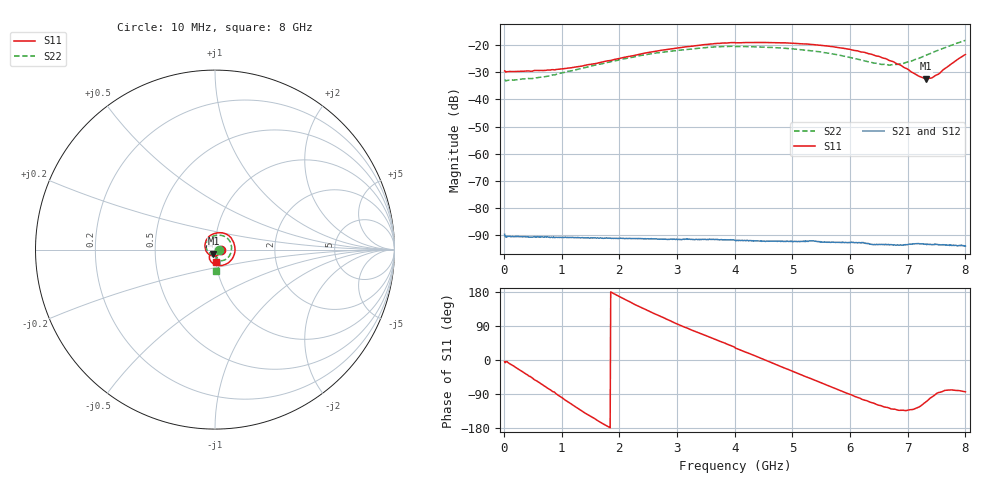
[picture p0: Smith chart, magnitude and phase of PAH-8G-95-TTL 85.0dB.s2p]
! MTS Systemtechnik GmbH
! S-Parameters
! Model: PAH-8G/95-TTL
! Attenuation Step: 85.0dB
! Rohde & Schwarz ZVB8 2Ports - Version 4.11 - 1145.1010k08 SN: 100119
! S2P File Measurements:
! S11 S21 S12 S22
# HZ  S  DB  R  50.00
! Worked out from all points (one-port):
!   800 points, 10 MHz to 8 GHz, reference 50 ohm
!   lowest |S11| = -32.3 dB at 7.32 GHz (marker M1), VSWR 1.05, Z = 49.1 - j2.23 ohm
!   |S11| at or under -10 dB: start of sweep to end of sweep
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1e7  -29.49 -3.7  -89.57 -1.8  -89.72 0.8  -32.75 -5.0
2e8  -29.70 -19.4  -90.45 -28.3  -90.44 -28.0  -32.80 -23.8
6.8e8  -29.35 -66.5  -90.59 -94.7  -90.57 -94.8  -31.70 -79.9
1.02e9  -28.76 -101.1  -90.67 -141.3  -90.71 -141.3  -30.18 -117.2
1.35e9  -27.72 -134.8  -90.86 173.2  -90.80 173.1  -28.55 -149.8
2.05e9  -24.64 163.6  -91.12 76.8  -91.16 76.9  -25.16 151.5
2.68e9  -22.09 117.0  -91.38 -10.4  -91.35 -10.0  -22.81 107.4
3.43e9  -19.94 68.8  -91.49 -111.8  -91.58 -112.0  -21.05 59.9
4.01e9  -19.17 31.5  -91.87 166.0  -91.86 166.8  -20.54 24.6
4.64e9  -19.06 -7.2  -92.09 80.9  -92.21 80.3  -20.86 -11.3
5.34e9  -19.79 -50.4  -92.03 -17.0  -92.04 -16.5  -22.11 -48.3
5.76e9  -20.79 -75.9  -92.54 -74.6  -92.69 -74.7  -23.47 -66.8
6.11e9  -22.03 -97.5  -92.65 -124.7  -92.71 -123.4  -25.07 -77.8
6.41e9  -23.70 -113.9  -93.41 -166.3  -93.52 -166.9  -26.59 -81.0
6.67e9  -25.57 -126.4  -93.31 159.1  -93.39 159.7  -27.36 -76.6
6.93e9  -28.17 -132.9  -93.60 125.4  -93.67 126.1  -26.71 -70.1
7.18e9  -31.33 -125.1  -93.05 90.4  -93.14 91.0  -24.98 -66.1
7.32e9  -32.31 -110.2  -93.25 69.5  -93.21 68.7  -23.71 -66.8
7.41e9  -32.12 -98.6  -93.42 57.0  -93.42 57.5  -22.98 -67.9
7.52e9  -30.82 -86.7  -93.38 41.6  -93.44 41.4  -22.01 -69.9
7.85e9  -25.43 -80.3  -93.80 -4.0  -93.95 -4.2  -19.33 -81.0
8e9  -23.47 -84.0  -93.98 -26.1  -93.72 -26.7  -18.29 -87.3
